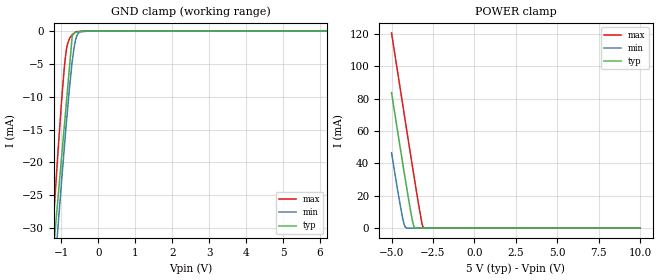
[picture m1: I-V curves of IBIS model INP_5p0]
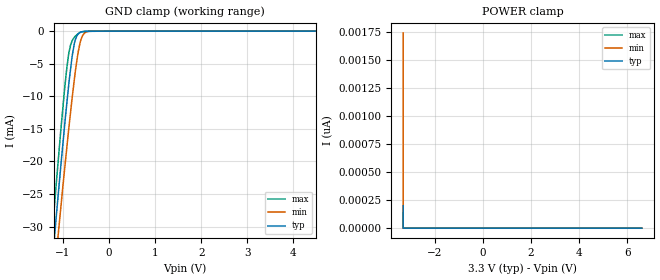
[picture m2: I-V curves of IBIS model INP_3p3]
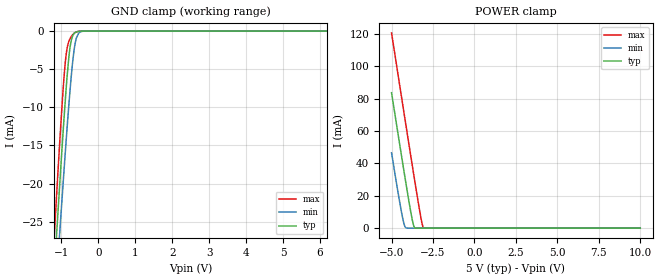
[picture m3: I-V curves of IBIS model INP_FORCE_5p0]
[IBIS Ver]   3.2
[Comment char]  |_char
[File Name]   trs3221e_rgt.ibs
[File Rev]   1.0 | x_die
[Date]   November 18, 2020
[Source]   Data created from TI-SPICE simulations at TI-SLL.
[Notes]   The following is an IBIS list for TRS3221E RGT
[Disclaimer] Property of Texas Instruments Incorporated.  Unauthorized
   reproduction and/or distribution is strictly prohibited.
   This product is protected under copyright law.
   Created  2020, (C) Copyright  2020, Texas Instruments
   Incorporated, All Rights Reserved
   UNLESS THERE IS A SIGNED, WRITTEN AGREEMENT TO THE
   CONTRARY, TEXAS INSTRUMENTS (TI) IS PROVIDING THE IBIS
   MODELS  AND WITHOUT ANY WARRANTY, EXPRESSED OR
   IMPLIED.  TI assumes no liability for:
   1) the accuracy of the IBIS models provided to your
   company;
   2) the proper functioning of these IBIS Models in your
   design or for any resulting applications; or
   3) infringement of patents, copyrights or intellectual
   property rights resulting from your use of these IBIS
   models.
   TI provides IBIS Models as a service to our customers.
   You and your company shall not distribute, sell or give
   these models to anyone else without prior written
   permission from TI.
   TI reserves the right to make changes to our products or
   to discontinue any semiconductor product or service
   without notice, and advises our customers to obtain the
   latest version of relevant information to verify, before
   placing orders, that the information being relied on is
   current.
   Please be aware that your receipt and use of the IBIS
   information provided shall serve as acceptance of these
   terms and conditions.  If you do not accept these terms,
   you should return or destroy the IBIS models and any
   other accompanying information immediately.
| Component TRS3221E RGT
[Component]   TRS3221E_RGT
[Manufacturer]   Texas Instruments, Inc.
[Package]   |QFN (RGT) 16-pin
|   typ   min   max
R_pkg   0.0658   0.0248   0.0806
L_pkg   0.8404nH   0.6985nH   1.0659nH
C_pkg   0.1111pF   0.1026pF   0.1480pF
[Pin]   signal_name   model_name   R_pin   L_pin   C_pin
1   ENB   INP   na   na   na
2   C1P   NC   na   na   na
3   VPLUS   NC   na   na   na
4   C1N   NC   na   na   na
5   C2P   NC   na   na   na
6   C2N   NC   na   na   na
7   VMINUS   NC   na   na   na
8   RIN   RIN   na   na   na
9   ROUT   ROUT   na   na   na
10   INVALIDB   INVALIDB   na   na   na
11   DIN   INP   na   na   na
12   FORCEON   INP_FORCE   na   na   na
13   DOUT   DOUT   na   na   na
14   GND   GND   na   na   na
15   VCC   POWER   na   na   na
16   FORCEOFFB   INP_FORCE   na   na   na
| Model INP
[Model Selector]   INP
INP_5p0   5 volt Vcc
INP_3p3   3.3 volt Vcc
| Model INP_FORCE
[Model Selector]   INP_FORCE
INP_FORCE_5p0   5 volt Vcc
INP_FORCE_3p3   3.3 volt Vcc
| Model INVALIDB
[Model Selector]   INVALIDB
INVALIDB_5p0   5 volt Vcc
INVALIDB_3p3   3.3 volt Vcc
| Model RIN
[Model Selector]   RIN
RIN_5p0   5 volt Vcc
RIN_3p3   3.3 volt Vcc
| Model ROUT
[Model Selector]   ROUT
ROUT_5p0   5 volt Vcc
ROUT_3p3   3.3 volt Vcc
| Model DOUT
[Model Selector]   DOUT
DOUT_5p0   5 volt Vcc
DOUT_3p3   3.3 volt Vcc
| Models and submodels in the file (12): INP_5p0 (Input), INP_3p3 (Input), INP_FORCE_5p0 (Input), INP_FORCE_3p3 (Input), INVALIDB_5p0 (Output), INVALIDB_3p3 (Output), RIN_5p0 (Input), RIN_3p3 (Input), ROUT_5p0 (3-state), ROUT_3p3 (3-state), DOUT_5p0 (3-state), DOUT_3p3 (3-state)
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[Model]   INP_5p0
Model_type   Input
Vinl = 0.8
Vinh = 2.4
|   typ   min   max
C_comp   0.75pF   0.72pF   0.79pF
[Voltage Range]   5   4.5   5.5
[Temperature Range]   27   110   -40
[Power Clamp Reference]   5   4.5   5.5
[GND Clamp Reference]   0   0   0
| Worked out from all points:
|   GND clamp passes 1 mA (typ) near -0.71 V on its own axis
|   POWER clamp passes 1 mA (typ) near -3.64 V on its own axis
[GND Clamp]
|   Voltage   I(typ)   I(min)   I(max)
-5V       -353.7mA   -333.1mA   -374.3mA
-1.343V   -44.3mA    -48.78mA   -40.41mA
-1.219V   -34.23mA   -39.59mA   -29.6mA
-1.161V   -30.19mA   -35.23mA   -24.64mA
-1.069V   -24.33mA   -28.57mA   -16.92mA
-884.1mV  -12.43mA   -15.57mA   -3.834mA
-824.5mV  -8.612mA   -11.7mA    -1.87mA
-702.6mV  -786.6uA   -4.649mA   -549.9uA
-611.8mV  -189.5uA   -1.343mA   -150.9uA
-513.5mV  -98.53uA   -211.2uA   -55.81uA
-284.9mV  -2.302uA   -935.4nA   -369.7nA
10V       0A         0A         0A
[POWER Clamp]
|   Voltage   I(typ)   I(min)   I(max)
-5V       83.65mA    46.54mA    120.6mA
-4.452V   48.08mA    12.84mA    84.53mA
-4.334V   40.54mA    6.495mA    76.82mA
-4.221V   33.3mA     1.772mA    69.38mA
-4.113V   26.49mA    140.8uA    62.32mA
-3.842V   10.11mA    164.9nA    44.74mA
-3.654V   1.221mA    38.71nA    32.63mA
-3.565V   74.33uA    0A         26.92mA
-3.242V   129.3nA    0A         7.188mA
-3.129V   0A         0A         1.622mA
-3.071V   0A         0A         250.9uA
10V       0A         0A         0A
[Model]   INP_3p3
Model_type   Input
Vinl = 0.8
Vinh = 2.0
|   typ   min   max
C_comp   0.80pF   0.77pF   0.84pF
[Voltage Range]   3.3   3   3.6
[Temperature Range]   27   110   -40
[Power Clamp Reference]   3.3   3   3.6
[GND Clamp Reference]   0   0   0
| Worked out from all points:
|   GND clamp passes 1 mA (typ) near -0.71 V on its own axis
[GND Clamp]
|   Voltage   I(typ)   I(min)   I(max)
-3.3V     -208.9mA   -199.9mA   -218.1mA
-1.249V   -36.59mA   -41.76mA   -32.16mA
-1.188V   -31.75mA   -37.27mA   -26.96mA
-1.15V    -28.66mA   -34.48mA   -23.64mA
-1.051V   -20.9mA    -27.29mA   -15.42mA
-962.6mV  -14.25mA   -20.98mA   -8.635mA
-879mV    -8.425mA   -15.25mA   -3.604mA
-756.1mV  -1.97mA    -7.529mA   -967.5uA
-631.4mV  -227.7uA   -1.828mA   -207.9uA
-547.4mV  -50.67uA   -412.4uA   -55.6uA
-430.7mV  -39.29uA   -32.69uA   -11.7uA
6.6V      0A         0A         0A
[POWER Clamp]
|   Voltage   I(typ)   I(min)   I(max)
-3.3V     199.5pA    1.746nA    133.2pA
-3.3V     0A         0A         0A
-3.3V     0A         0A         0A
6.6V      0A         0A         0A
[Model]   INP_FORCE_5p0
Model_type   Input
Vinl = 0.8
Vinh = 2.4
|   typ   min   max
C_comp   0.748pF	0.718pF	0.787pF
[Voltage Range]   5   4.5   5.5
[Temperature Range]   27   110   -40
[Power Clamp Reference]   5   4.5   5.5
[GND Clamp Reference]   0   0   0
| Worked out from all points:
|   GND clamp passes 1 mA (typ) near -0.71 V on its own axis
|   POWER clamp passes 1 mA (typ) near -3.64 V on its own axis
[GND Clamp]
|   Voltage   I(typ)   I(min)   I(max)
-5V       -353.7mA   -333.1mA   -374.3mA
-1.235V   -35.47mA   -40.72mA   -30.95mA
-1.13V    -27.08mA   -32.97mA   -21.96mA
-1.115V   -25.89mA   -31.88mA   -20.7mA
-1.04V    -20.05mA   -26.44mA   -14.54mA
-950mV    -13.31mA   -20.07mA   -7.751mA
-875mV    -8.109mA   -14.94mA   -3.428mA
-740mV    -1.507mA   -6.554mA   -809.1uA
-650mV    -310.9uA   -2.413mA   -275.2uA
-590mV    -107.9uA   -908.6uA   -102.9uA
-305mV    -239.7nA   -1.528uA   -42.87nA
10V       0A         0A         0A
[POWER Clamp]
|   Voltage   I(typ)   I(min)   I(max)
-5V       83.65mA    46.54mA    120.6mA
-4.505V   51.49mA    15.9mA     88.01mA
-4.325V   39.93mA    6.032mA    76.21mA
-4.205V   32.29mA    1.341mA    68.35mA
-4.115V   26.63mA    150.8uA    62.47mA
-3.845V   10.27mA    24.31nA    44.91mA
-3.665V   1.54mA     0A         33.31mA
-3.575V   108.8uA    0A         27.57mA
-3.215V   0A         0A         5.682mA
-3.125V   0A         0A         1.482mA
-3.065V   0A         0A         195.5uA
10V       0A         0A         0A
